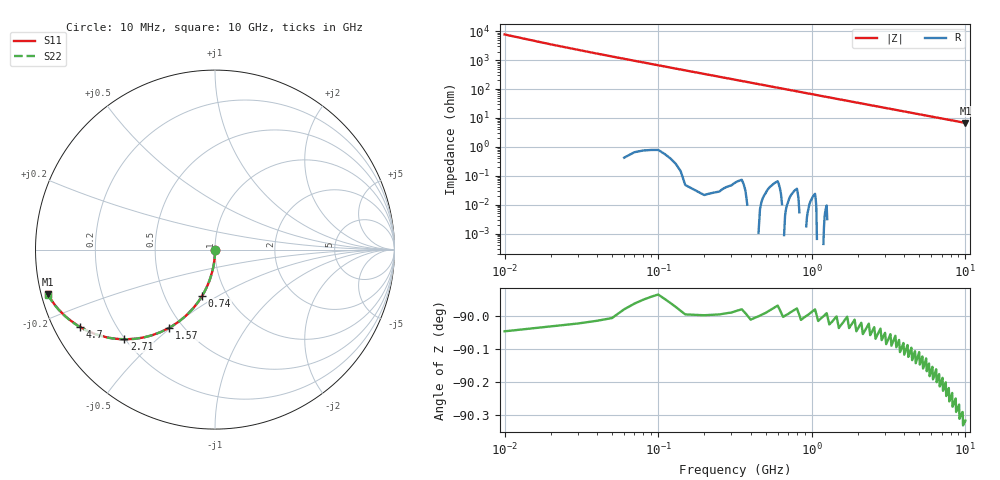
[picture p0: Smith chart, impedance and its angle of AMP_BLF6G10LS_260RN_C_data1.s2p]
! Created Mon Mar 29 11:07:01 2010
# ghz S ma R 50
! 2 Port Network Data from SP1.SP block
! freq  magS11  angS11  magS21  angS21  magS12  angS12  magS22  angS22
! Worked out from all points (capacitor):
!   1000 points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, 10 MHz to 10 GHz, reference 50 ohm
!   read as one part in shunt: C = 2.37 pF near 60 MHz
!   lowest |Z| = 6.76 ohm at 10 GHz (marker M1)
!   S11 on the Smith chart (normalised r, x): 10 MHz: 1.00, -0.01; 740 MHz: 0.77, -0.42; 1.57 GHz: 0.42, -0.49; 2.71 GHz: 0.20, -0.40; 4.7 GHz: 0.08, -0.26; 10 GHz: 0.02, -0.13
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0.01  0.003222 -89.8  1 -0.2  1 -0.2  0.003145 -89.8
0.04  0.01457 -90.7  0.9999 -0.8  0.9999 -0.8  0.01477 -90.7
0.07  0.02566 -91.5  0.9996 -1.5  0.9996 -1.5  0.02607 -91.4
0.09  0.03297 -91.9  0.9994 -1.9  0.9994 -1.9  0.0335 -91.9
0.11  0.0406 -92.4  0.9991 -2.4  0.9991 -2.4  0.04096 -92.3
0.14  0.05252 -93.0  0.9986 -3.0  0.9986 -3.0  0.05218 -93.0
0.2  0.07463 -94.2  0.9972 -4.3  0.9972 -4.3  0.07434 -94.3
0.29  0.1072 -96.2  0.9942 -6.2  0.9942 -6.2  0.1074 -96.2
0.41  0.1516 -98.7  0.9884 -8.7  0.9884 -8.7  0.1511 -98.7
0.56  0.2038 -101.8  0.9788 -11.8  0.9788 -11.8  0.2043 -101.8
0.74  0.2657 -105.5  0.9639 -15.4  0.9639 -15.4  0.2657 -105.4
1.12  0.3854 -112.7  0.9227 -22.7  0.9227 -22.7  0.3851 -112.7
1.57  0.5051 -120.4  0.863 -30.4  0.863 -30.4  0.5048 -120.3
1.68  0.5301 -122.1  0.8475 -32.1  0.8475 -32.1  0.5305 -122.1
2.17  0.629 -129.0  0.7776 -39.0  0.7776 -39.0  0.6285 -129.0
2.71  0.7103 -135.3  0.7038 -45.4  0.7038 -45.4  0.7103 -135.3
3.34  0.7794 -141.3  0.6266 -51.3  0.6266 -51.3  0.7793 -141.2
4.7  0.8678 -150.4  0.4966 -60.4  0.4966 -60.4  0.8681 -150.3
5.01  0.8809 -151.9  0.473 -62.0  0.473 -62.0  0.8812 -151.8
6.67  0.9271 -158.2  0.3745 -68.3  0.3745 -68.3  0.9274 -158.0
8.34  0.9514 -162.3  0.3079 -72.5  0.3079 -72.5  0.9516 -162.1
10  0.965 -165.2  0.2611 -75.4  0.2611 -75.4  0.9655 -164.9
